(* Logix 5000 AddOnInstructionDefinition export BMC_AOI_PROC_BAE00LC; software revision 20.04 *)

TYPE BMC_UDT_PROC_BAE00LC_Data_5117US :   // BAE00LC Process Data
STRUCT
   I : BMC_UDT_PROC_BAE00LC_Inputs_5117US;
   IOL_Diag : BMC_UDT_DIAG_IOL_Data_1916US;
END_STRUCT
END_TYPE

TYPE IO_Link_Port_Data :
STRUCT
   Inputs : SINT[48];
   Outputs : SINT[48];
END_STRUCT
END_TYPE

TYPE BMC_UDT_DIAG_IOL_Data_1916US :   // IO-Link Diagnostics
STRUCT
   DeviceOK : BOOL;
   MismatchFault : BOOL;
   CommFault : BOOL;
   ValidationFailed : BOOL;
   ProcessDataInvalid : BOOL;
   DSValidationFailure : BOOL;
   IOLShortCircuit : BOOL;
   Event : BMC_UDT_DIAG_IOL_Event_1916US[3];
   VendorID : SINT[2];
   DeviceID : SINT[3];
END_STRUCT
END_TYPE

TYPE BMC_UDT_PROC_BAE00LC_Inputs_5117US :   // BAE00LC Input Data
STRUCT
   Value : INT;   // Process Value
   BDC1 : BOOL;   // Switch Point 1
END_STRUCT
END_TYPE

TYPE BMC_UDT_DIAG_IOL_Event_1916US :   // IO-Link Event Codes
STRUCT
   Code : SINT;
   Additional_Data_1 : SINT;
   Additional_Data_2 : SINT;
END_STRUCT
END_TYPE

ADD_ON_INSTRUCTION BMC_AOI_PROC_BAE00LC   (* revision 4.0 3C0718US, vendor Balluff, Inc. *)
// BAE SA-CS-027-YI-BPxx,x-GS04
// H1.0 S1.0
// Revision note:
// Initial Release
VAR_IN_OUT
   IO_Link_Port_Data : IO_Link_Port_Data; {required}
   Mapped_BAE00LC_Data : BMC_UDT_PROC_BAE00LC_Data_5117US; {required}
END_VAR

ROUTINE Logic   (* ladder *)
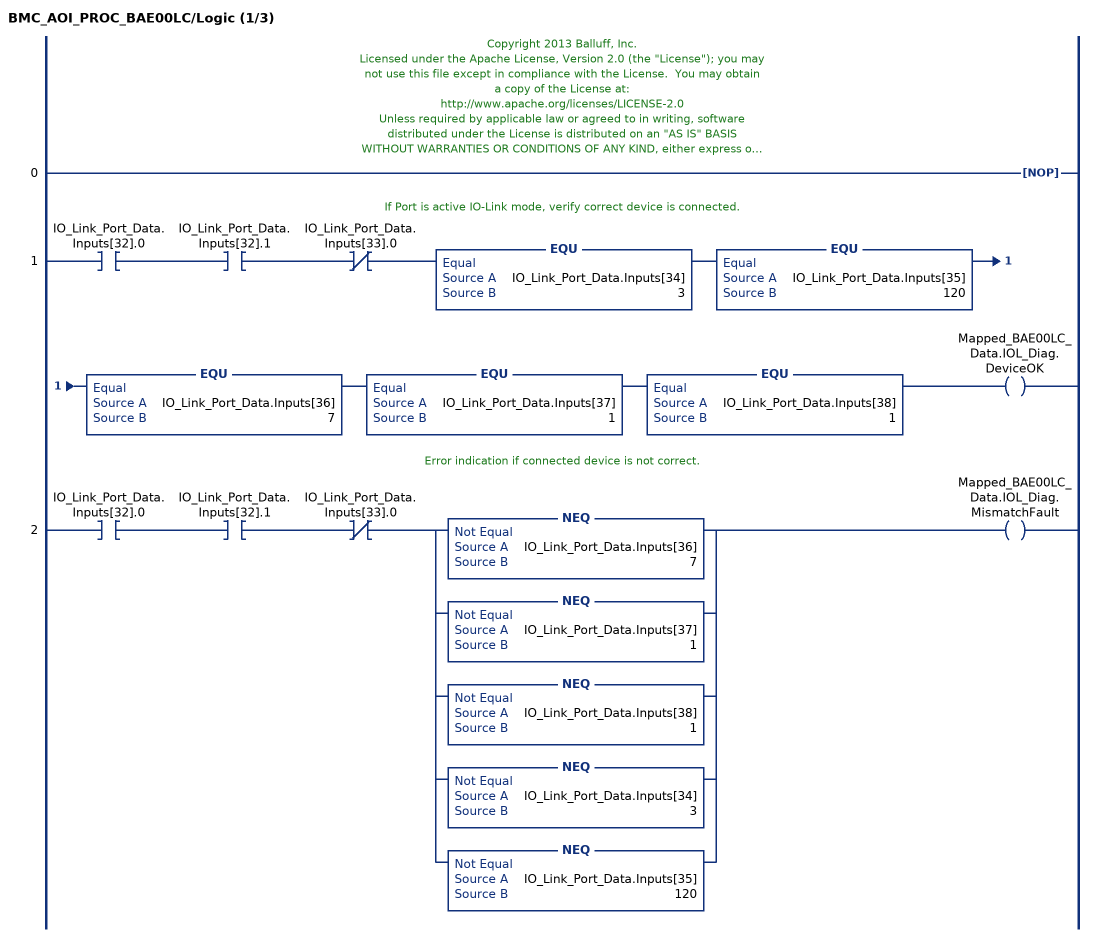
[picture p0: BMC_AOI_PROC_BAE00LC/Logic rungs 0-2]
   // Copyright 2013 Balluff, Inc.
   // Licensed under the Apache License, Version 2.0 (the "License"); you may
   // not use this file except in compliance with the License.  You may obtain
   // a copy of the License at:
   // http://www.apache.org/licenses/LICENSE-2.0
   // Unless required by applicable law or agreed to in writing, software
   // distributed under the License is distributed on an "AS IS" BASIS
   // WITHOUT WARRANTIES OR CONDITIONS OF ANY KIND, either express or
   // implied.  See the License for the specific language governing
   // permissions and limitations under the License.
   0: NOP();
   // If Port is active IO-Link mode, verify correct device is connected.
   1: XIC(IO_Link_Port_Data.Inputs[32].0)XIC(IO_Link_Port_Data.Inputs[32].1)XIO(IO_Link_Port_Data.Inputs[33].0)EQU(IO_Link_Port_Data.Inputs[34],3)EQU(IO_Link_Port_Data.Inputs[35],120)EQU(IO_Link_Port_Data.Inputs[36],7)EQU(IO_Link_Port_Data.Inputs[37],1)EQU(IO_Link_Port_Data.Inputs[38],1)OTE(Mapped_BAE00LC_Data.IOL_Diag.DeviceOK);
   // Error indication if connected device is not correct.
   2: XIC(IO_Link_Port_Data.Inputs[32].0)XIC(IO_Link_Port_Data.Inputs[32].1)XIO(IO_Link_Port_Data.Inputs[33].0)[NEQ(IO_Link_Port_Data.Inputs[36],7) ,NEQ(IO_Link_Port_Data.Inputs[37],1) ,NEQ(IO_Link_Port_Data.Inputs[38],1) ,NEQ(IO_Link_Port_Data.Inputs[34],3) ,NEQ(IO_Link_Port_Data.Inputs[35],120) ]OTE(Mapped_BAE00LC_Data.IOL_Diag.MismatchFault);
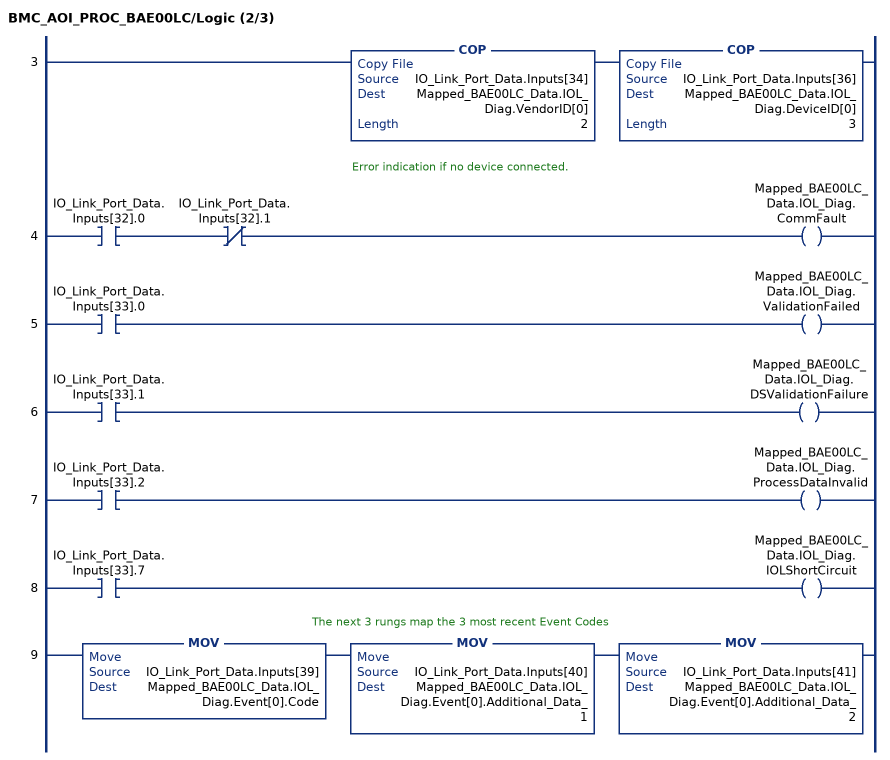
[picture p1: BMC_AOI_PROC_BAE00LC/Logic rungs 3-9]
   3: COP(IO_Link_Port_Data.Inputs[34],Mapped_BAE00LC_Data.IOL_Diag.VendorID[0],2)COP(IO_Link_Port_Data.Inputs[36],Mapped_BAE00LC_Data.IOL_Diag.DeviceID[0],3);
   // Error indication if no device connected.
   4: XIC(IO_Link_Port_Data.Inputs[32].0)XIO(IO_Link_Port_Data.Inputs[32].1)OTE(Mapped_BAE00LC_Data.IOL_Diag.CommFault);
   5: XIC(IO_Link_Port_Data.Inputs[33].0)OTE(Mapped_BAE00LC_Data.IOL_Diag.ValidationFailed);
   6: XIC(IO_Link_Port_Data.Inputs[33].1)OTE(Mapped_BAE00LC_Data.IOL_Diag.DSValidationFailure);
   7: XIC(IO_Link_Port_Data.Inputs[33].2)OTE(Mapped_BAE00LC_Data.IOL_Diag.ProcessDataInvalid);
   8: XIC(IO_Link_Port_Data.Inputs[33].7)OTE(Mapped_BAE00LC_Data.IOL_Diag.IOLShortCircuit);
   // The next 3 rungs map the 3 most recent Event Codes
   9: MOV(IO_Link_Port_Data.Inputs[39],Mapped_BAE00LC_Data.IOL_Diag.Event[0].Code)MOV(IO_Link_Port_Data.Inputs[40],Mapped_BAE00LC_Data.IOL_Diag.Event[0].Additional_Data_1)MOV(IO_Link_Port_Data.Inputs[41],Mapped_BAE00LC_Data.IOL_Diag.Event[0].Additional_Data_2);
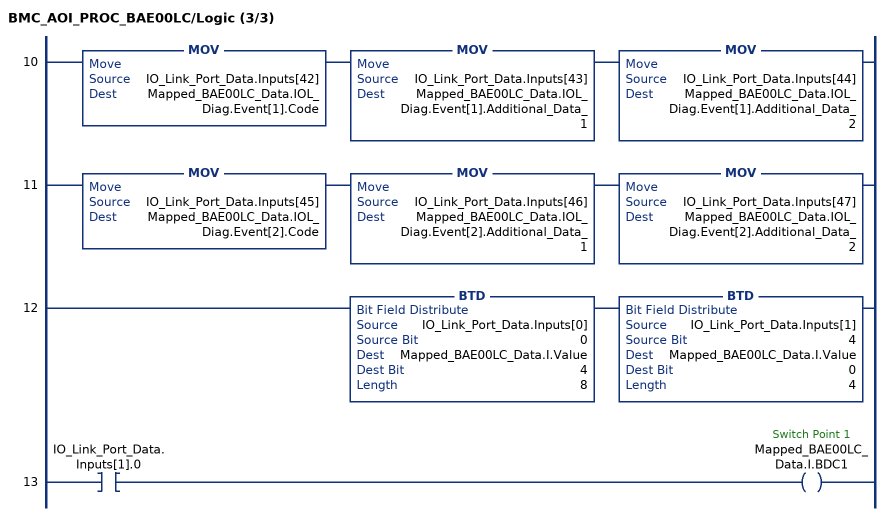
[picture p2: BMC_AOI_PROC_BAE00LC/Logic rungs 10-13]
   10: MOV(IO_Link_Port_Data.Inputs[42],Mapped_BAE00LC_Data.IOL_Diag.Event[1].Code)MOV(IO_Link_Port_Data.Inputs[43],Mapped_BAE00LC_Data.IOL_Diag.Event[1].Additional_Data_1)MOV(IO_Link_Port_Data.Inputs[44],Mapped_BAE00LC_Data.IOL_Diag.Event[1].Additional_Data_2);
   11: MOV(IO_Link_Port_Data.Inputs[45],Mapped_BAE00LC_Data.IOL_Diag.Event[2].Code)MOV(IO_Link_Port_Data.Inputs[46],Mapped_BAE00LC_Data.IOL_Diag.Event[2].Additional_Data_1)MOV(IO_Link_Port_Data.Inputs[47],Mapped_BAE00LC_Data.IOL_Diag.Event[2].Additional_Data_2);
   12: BTD(IO_Link_Port_Data.Inputs[0],0,Mapped_BAE00LC_Data.I.Value,4,8)BTD(IO_Link_Port_Data.Inputs[1],4,Mapped_BAE00LC_Data.I.Value,0,4);
   13: XIC(IO_Link_Port_Data.Inputs[1].0)OTE(Mapped_BAE00LC_Data.I.BDC1);
END_ROUTINE
END_ADD_ON_INSTRUCTION
